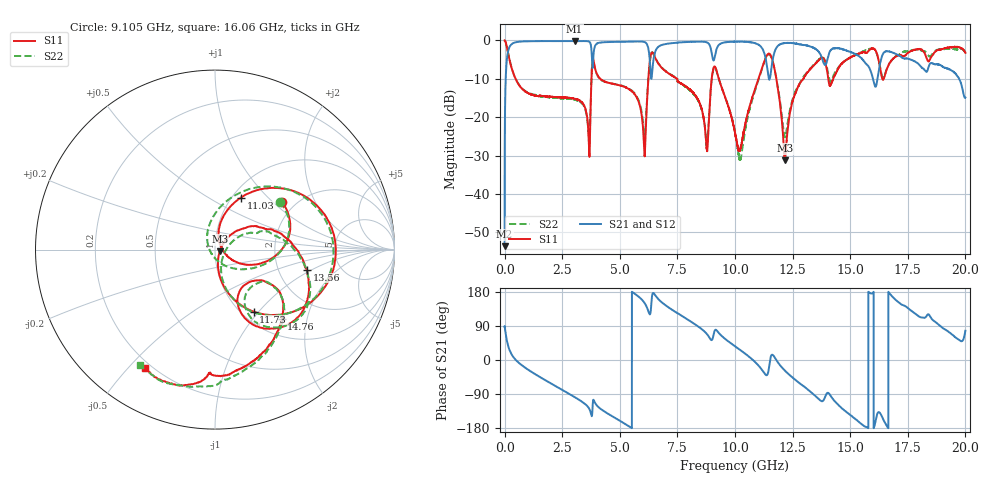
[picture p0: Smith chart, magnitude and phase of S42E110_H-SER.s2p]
! Created Wed Nov 25 21:55:14 2020
# khz S ma R 50
! 2 Port Network Data from SP1.SP block
! freq  magS11  angS11  magS21  angS21  magS12  angS12  magS22  angS22
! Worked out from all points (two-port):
!   20001 points, 300 kHz to 20 GHz, reference 50 ohm
!   highest |S21| = -0.15 dB at 3.038 GHz (marker M1); lowest = -53.6 dB at 300 kHz (marker M2)
!   |S21| within 3 dB of the highest: 140.2 MHz to 3.777 GHz (3.637 GHz wide, 186 % of centre); 6.525 GHz to 8.984 GHz (2.459 GHz wide, 31.7 % of centre)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
!   lowest |S11| = -31.2 dB at 12.17 GHz (marker M3), VSWR 1.06, Z = 52.7 - j0.914 ohm
!   |S11| at or under -10 dB: 475.1 MHz to 3.77 GHz (3.295 GHz wide, 155 % of centre); 4.149 GHz to 6.24 GHz (2.091 GHz wide, 40.2 % of centre); 9.3 GHz to 11.02 GHz (1.718 GHz wide, 16.9 % of centre)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
!   |S22| runs from -31.2 to 0.0 dB; largest |S21 - S12| = 0.019
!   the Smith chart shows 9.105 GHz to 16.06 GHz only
!   S11 on the Smith chart (normalised r, x): 9.105 GHz: 1.69, +1.14; 11.03 GHz: 1.10, +0.71; 11.73 GHz: 1.13, -0.94; 13.56 GHz: 2.89, -0.89; 14.76 GHz: 1.30, -1.42; 16.06 GHz: 0.17, -0.56
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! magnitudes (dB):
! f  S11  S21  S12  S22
! 300 kHz  0.0  -53.6  -53.5  0.0
! 106.3 MHz  -1.9  -4.5  -4.5  -1.9
! 248.3 MHz  -5.9  -1.3  -1.3  -5.9
! 3.038 GHz  -15.2  -0.2  -0.2  -15.4
! 3.334 GHz  -16.0  -0.2  -0.2  -16.2
! 3.643 GHz  -24.6  -0.2  -0.2  -24.6
! 3.885 GHz  -6.0  -2.3  -2.3  -6.1
! 6.055 GHz  -27.7  -0.4  -0.4  -24.1
! 6.346 GHz  -3.8  -9.0  -9.0  -3.7
! 6.667 GHz  -6.0  -1.7  -1.7  -5.9
! 8.762 GHz  -27.7  -0.5  -0.5  -27.1
! 9.105 GHz  -6.8  -4.8  -4.7  -6.9
! 10 GHz  -24.1  -0.3  -0.3  -23.8
! 11.03 GHz  -9.8  -1.1  -1.2  -10.1
! 11.73 GHz  -7.8  -2.8  -2.8  -7.8
! 12.17 GHz  -31.2  -0.7  -0.7  -25.1
! 13.33 GHz  -7.1  -1.7  -1.7  -6.9
! 13.56 GHz  -5.6  -2.5  -2.4  -5.5
! 14.76 GHz  -5.4  -2.5  -2.4  -5.4
! 16.06 GHz  -2.3  -11.7  -11.7  -2.3
! 16.67 GHz  -6.4  -2.8  -3.0  -6.3
! 20 GHz  -3.3  -14.8  -14.8  -3.1
